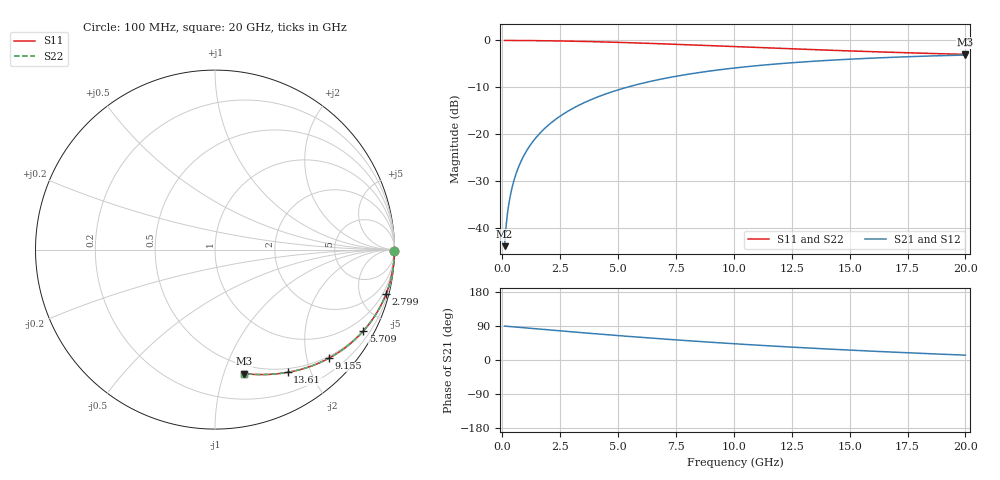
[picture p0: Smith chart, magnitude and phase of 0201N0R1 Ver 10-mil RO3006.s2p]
# GHz S MA R 50
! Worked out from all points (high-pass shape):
!   1601 points, 100 MHz to 20 GHz, reference 50 ohm
!   highest |S21| = -3.11 dB at 20 GHz (marker M1); lowest = -44.0 dB at 100 MHz (marker M2)
!   |S21| within 3 dB of the highest: 9.636 GHz to end of sweep
!   lowest |S11| = -3.0 dB at 20 GHz (marker M3), VSWR 5.90, Z = 21 - j58.6 ohm
!   |S11| at or under -10 dB: nowhere
!   |S22| runs from -3.0 to 0.0 dB; largest |S21 - S12| = 0
!   S11 on the Smith chart (normalised r, x): 100 MHz: open; 2.799 GHz: 0.48, -7.78; 5.709 GHz: 0.47, -3.84; 9.155 GHz: 0.46, -2.42; 13.61 GHz: 0.45, -1.66; 20 GHz: 0.42, -1.17
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0.1  1 -0.5  0.006318 89.5  0.006318 89.5  1 -0.5
0.14975  1 -0.8  0.00946 89.2  0.00946 89.2  1 -0.8
0.224375  0.9999 -1.2  0.01417 88.8  0.01417 88.8  0.9999 -1.2
0.274125  0.9998 -1.4  0.01731 88.6  0.01731 88.6  0.9998 -1.4
0.3985  0.9997 -2.1  0.02516 87.9  0.02516 87.9  0.9997 -2.1
0.4855625  0.9995 -2.6  0.03066 87.4  0.03066 87.4  0.9995 -2.6
0.5975  0.9993 -3.1  0.03771 86.8  0.03771 86.8  0.9993 -3.1
0.871125  0.9985 -4.6  0.05492 85.4  0.05492 85.4  0.9985 -4.6
1.219375  0.997 -6.4  0.07672 83.6  0.07672 83.6  0.997 -6.4
1.654688  0.9945 -8.7  0.1038 81.3  0.1038 81.3  0.9945 -8.7
2.177062  0.9906 -11.4  0.1358 78.6  0.1358 78.6  0.9906 -11.4
2.798938  0.9847 -14.6  0.1731 75.4  0.1731 75.4  0.9847 -14.6
3.420812  0.9776 -17.7  0.2095 72.2  0.2095 72.2  0.9776 -17.7
4.478  0.9629 -23.0  0.2685 67.0  0.2685 67.0  0.9629 -23.0
5.709313  0.9426 -28.8  0.3321 61.1  0.3321 61.1  0.9426 -28.8
6.741625  0.9238 -33.5  0.3808 56.4  0.3808 56.4  0.9238 -33.5
9.1545  0.8768 -43.6  0.478 46.2  0.478 46.2  0.8768 -43.6
10.05  0.8593 -47.1  0.5084 42.7  0.5084 42.7  0.8593 -47.1
13.37081  0.7988 -58.6  0.5978 31.1  0.5978 31.1  0.7988 -58.6
13.60712  0.7948 -59.4  0.6029 30.4  0.6029 30.4  0.7948 -59.4
16.69162  0.7486 -68.4  0.6583 21.3  0.6583 21.3  0.7486 -68.4
20  0.71 -76.8  0.6988 12.8  0.6988 12.8  0.71 -76.8
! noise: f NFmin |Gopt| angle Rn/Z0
0.1  0.003641  0.9937  0.515  0.1328
2.301  0.006383  0.8845  7.707  0.01194
4.515  0.008958  0.8241  11.9  0.01058
6.729  0.01131  0.7867  15.55  0.01071
8.943  0.0135  0.7606  19.08  0.01112
11.14  0.01557  0.7412  22.56  0.01161
13.36  0.01758  0.7259  26.06  0.01211
15.57  0.01953  0.7137  29.54  0.01261
17.79  0.02143  0.7038  33.02  0.01308
20  0.02331  0.6957  36.48  0.01354
